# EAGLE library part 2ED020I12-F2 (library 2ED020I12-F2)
2ED020I12-F2 SOP65P1030X265-36_32N-V Dual IGBT Driver IC
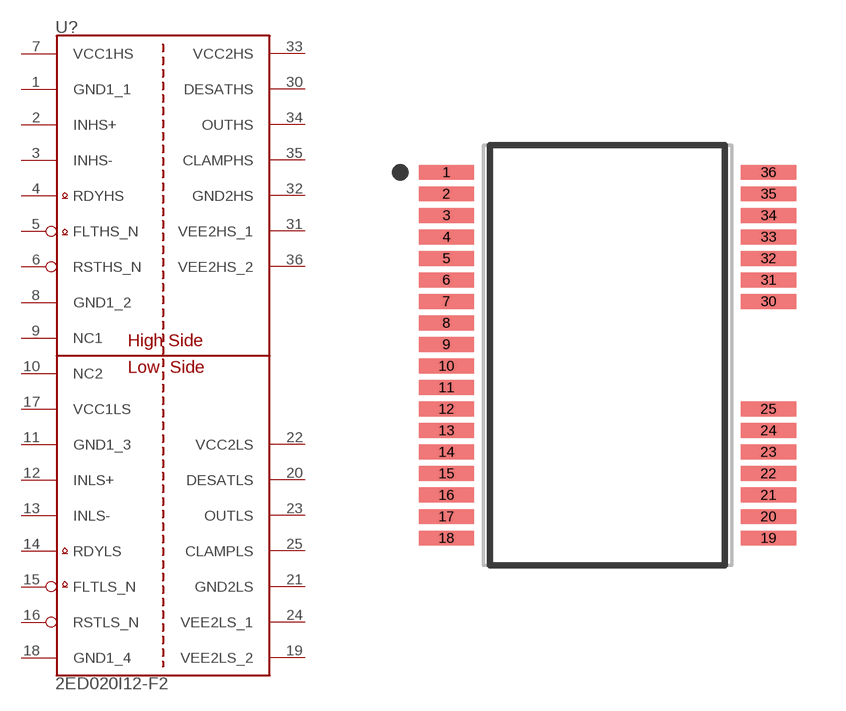
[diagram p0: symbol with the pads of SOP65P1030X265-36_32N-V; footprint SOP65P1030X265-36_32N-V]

Designator prefix U?

## 2ED020I12-F2  [SOP65P1030X265-36_32N-V]
1  GND1_1  pwr
2  INHS+  in
3  INHS-  in
4  RDYHS  oc
5  FLTHS_N  oc
6  RSTHS_N  in
7  VCC1HS  pwr
8  GND1_2  pwr
9  NC1  pas
10  NC2  pas
11  GND1_3  pwr
12  INLS+  in
13  INLS-  in
14  RDYLS  oc
15  FLTLS_N  oc
16  RSTLS_N  in
17  VCC1LS  pwr
18  GND1_4  pwr
19  VEE2LS_2  pwr
20  DESATLS  in
21  GND2LS  pwr
22  VCC2LS  pwr
23  OUTLS  out
24  VEE2LS_1  pwr
25  CLAMPLS  pas
30  DESATHS  in
31  VEE2HS_1  pwr
32  GND2HS  pwr
33  VCC2HS  pwr
34  OUTHS  out
35  CLAMPHS  pas
36  VEE2HS_2  pwr

## Footprint SOP65P1030X265-36_32N-V (pad centres in mm)
Original name SOP65P1030X265-36_32N-V Max Component Height - 2.65mm
smd 1.67 x 0.45: 1 -4.865,5.525; 2 -4.865,4.875; 3 -4.865,4.225; 4 -4.865,3.575; 5 -4.865,2.925; 6 -4.865,2.275; 7 -4.865,1.625; 8 -4.865,0.975; 9 -4.865,0.325; 10 -4.865,-0.325; 11 -4.865,-0.975; 12 -4.865,-1.625; 13 -4.865,-2.275; 14 -4.865,-2.925; 15 -4.865,-3.575; 16 -4.865,-4.225; 17 -4.865,-4.875; 18 -4.865,-5.525; 19 4.865,-5.525; 20 4.865,-4.875; 21 4.865,-4.225; 22 4.865,-3.575; 23 4.865,-2.925; 24 4.865,-2.275; 25 4.865,-1.625; 30 4.865,1.625; 31 4.865,2.275; 32 4.865,2.925; 33 4.865,3.575; 34 4.865,4.225; 35 4.865,4.875; 36 4.865,5.525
